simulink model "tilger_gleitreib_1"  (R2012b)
settings: Solver=ode2  StartTime=0.0  StopTime=10.0  RelTol=1e-3
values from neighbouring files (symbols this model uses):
  k = 10    [coulomb_10.m]    (also in coulomb_11.m; diff_filter_1.m = 250; diff_filter_2.m = 250; dry_friction_1.m = 2200)
  m = 400    [coulomb_1.m]    (also in coulomb_10.m = 10; coulomb_11.m = 10; coulomb_2.m; coulomb_3.m)
  rg = 20    [tilger_gleitreib1.m]    (also in tilger_gleitreib2.m = 100; tilger_gleitreib21.m = 0.5; tilger_gleitreib3.m = 8,      m1 = 0.1)
  x0 = [1;0]*1e-2    [rad_aufhaeng_1.m]    (also in slip_stick_3_1.m = 0.1; slip_stick_3_11.m = 0.1; suspension_1.m = [1 1 1 1]'; tilger_gleitreib1.m = 0.2)

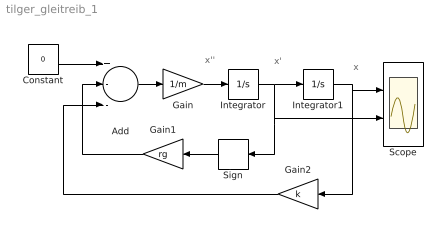
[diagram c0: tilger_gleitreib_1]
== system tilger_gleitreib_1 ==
  note: x
  note: x'
  note: x''
  Add : Sum  Inputs=+--
  Constant : Constant  Value=0
  Gain : Gain  Gain=1/m
  Gain1 : Gain  Gain=rg
  Gain2 : Gain  Gain=k
  Integrator : Integrator  ZeroCross=off
  Integrator1 : Integrator  InitialCondition=x0  ZeroCross=off
  Scope : Scope  NumInputPorts=2
  Sign : Signum
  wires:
  Constant/1 -> Add/1
  Add/1 -> Gain/1
  Gain/1 -> Integrator/1
  Gain1/1 -> Add/2
  Integrator1/1 -> Gain2/1, Scope/1
  Gain2/1 -> Add/3
  Integrator/1 -> Sign/1, Scope/2, Integrator1/1
  Sign/1 -> Gain1/1
